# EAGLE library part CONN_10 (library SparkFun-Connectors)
Multi connection point. Often used as Generic Header-pin footprint for 0.1 inch spaced/style header connections On any of the 0.1 inch spaced packages, you can populate with these: Break Away Headers - Straight (PRT-00116) Break Away Male Headers - Right Angle (PRT-00553) Female Headers (PRT-00115) Break Away Headers - Machine Pin (PRT-00117) Break Away Female Headers - Swiss Machine Pin (PRT-00743) Arduino Stackable Header - 10 Pin (PRT-11376) For SCREWTERMINALS and SPRING TERMINALS visit here: Screw Terimnals on SparkFun.com (5mm/3.5mm/2.54mm spacing) This device is also useful as a general connection point to wire up your design to another part of your project. Our various solder wires solder well into these plated through hole pads. Hook-Up Wire - Assortment (Stranded, 22 AWG) (PRT-11375) Hook-Up Wire - Assortment (Solid Core, 22 AWG) (PRT-11367) View the entire wire category on our website here Special notes: Molex polarized connector foot print use with SKU : PRT-08231 with associated crimp pins and housings. 1MM SMD Version SKU: PRT-10208 NOTES ON THE VARIANTS LOCK and LOCK_LONGPADS... This footprint was designed to help hold the alignment of a through-hole component (i.e. 6-pin header) while soldering it into place. You may notice that each hole has been shifted either up or down by 0.005 of an inch from it's more standard position (which is a perfectly straight line). This slight alteration caused the pins (the squares in the middle) to touch the edges of the holes.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
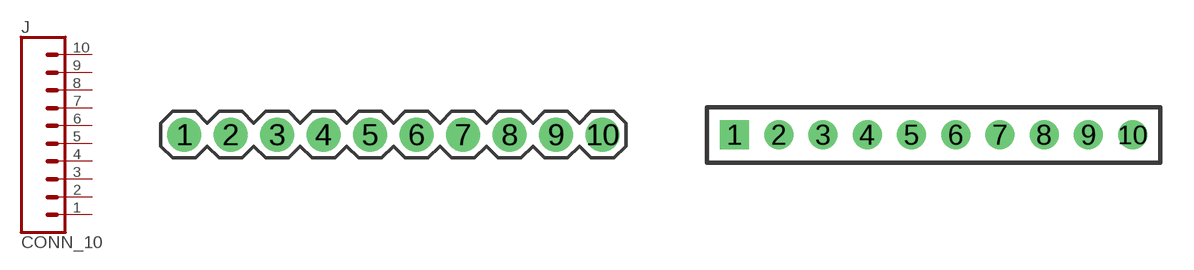
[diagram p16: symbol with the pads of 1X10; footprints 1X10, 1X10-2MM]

Designator prefix J

## CONN_10" (PROD_ID: CONN-11563)  [1X10]
1  1  pas
2  2  pas
3  3  pas
4  4  pas
5  5  pas
6  6  pas
7  7  pas
8  8  pas
9  9  pas
10  10  pas

## CONN_102MM (PROD_ID: CONN-08875; SF_ID: PRT-08272)  [1X10-2MM]
Pads as for 1X10

## CONN_102MMSMD (PROD_ID: CONN-09042; SF_ID: PRT-10030)  [1X10-2MM-SMD]
Pads as for 1X10

## CONN_10LOCK  [1X10_LOCK]
Pads as for 1X10

## CONN_10LOCK_LONGPADS  [1X10_LOCK_LONGPADS]
Pads as for 1X10

## CONN_10SMD_COMBO-FEMALE (PROD_ID: CONN-11219)  [1X10_SMD_COMBINED]
1A  1  pas
1B  1  pas
2A  2  pas
2B  2  pas
3A  3  pas
3B  3  pas
4A  4  pas
4B  4  pas
5A  5  pas
5B  5  pas
6A  6  pas
6B  6  pas
7A  7  pas
7B  7  pas
8A  8  pas
8B  8  pas
9A  9  pas
9B  9  pas
10A  10  pas
10B  10  pas

## CONN_10SMD_MALE (PROD_ID: CONN-11291)  [1X10_SMD_MALE]
Pads as for 1X10

## CONN_10NO_SILK_PTH_FEMALE (PROD_ID: CONN-11563)  [1X10_NO_SILK]
Pads as for 1X10

## CONN_10LOCK_NS  [1X10_LOCK_NS]
Pads as for 1X10

## CONN_101.25MM_SMD  [1X10-1.25MM-SMD]
Pads as for 1X10

## CONN_103.5MM-10  [SCREWTERMINAL-3.5MM-10]
Pads as for 1X10

## Footprint 1X10 (pad centres in mm)
Plated Through Hole -10 Pin Specifications: Pin count:10 Pin pitch:0.1" Example device(s): CONN_10
drill 1.016 pad 1.88: 1 0,0; 2 2.54,0; 3 5.08,0; 4 7.62,0; 5 10.16,0; 6 12.7,0; 7 15.24,0; 8 17.78,0; 9 20.32,0; 10 22.86,0

## Footprint 1X10-2MM (pad centres in mm)
Plated Through Hole -10 Pin 2mm Specifications: Pin count:10 Pin pitch:2mm Datasheet referenced for footprint Example device(s): CONN_10
drill 0.8 square: 1 0,0
drill 0.8: 2 2,0; 3 4,0; 4 6,0; 5 8,0; 6 10,0; 7 12,0; 8 14,0; 9 16,0; 10 18,0

## Footprint 1X10-2MM-SMD (pad centres in mm)
Plated Through Hole -10 Pin 2mm SMD Specifications: Pin count:10 Pin pitch:2mm Datasheet referenced for footprint Example device(s): CONN_10
smd 0.85 x 2.1: 1 0,-1.5; 2 2,1.5; 3 4,-1.5; 4 6,1.5; 5 8,-1.5; 6 10,1.5; 7 12,-1.5; 8 14,1.5; 9 16,-1.5; 10 18,1.5

## Footprint 1X10_LOCK (pad centres in mm)
Plated Through Hole -10 Pin Locking Footprint Holes are offset 0.005" to hold pins in place while soldering. Specifications: Pin count:10 Pin pitch:0.1" Example device(s): CONN_10
drill 1.016 pad 1.88: 1 0,0.127; 2 2.54,-0.127; 3 5.08,0.127; 4 7.62,-0.127; 5 10.16,0.127; 6 12.7,-0.127; 7 15.24,0.127; 8 17.78,-0.127; 9 20.32,0.127; 10 22.86,-0.127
